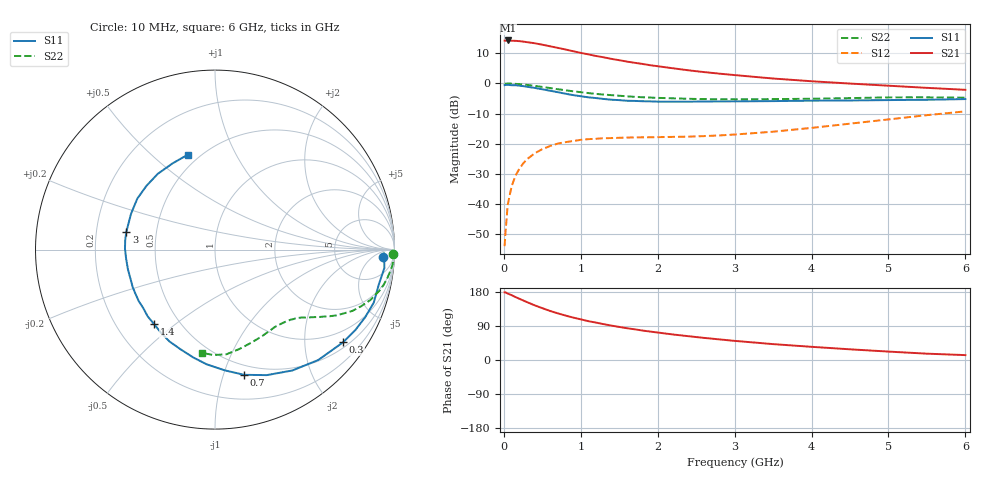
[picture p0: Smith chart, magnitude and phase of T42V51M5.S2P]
! Infineon Technologies  Discrete & RF Semiconductors
! BFR182T
! Si NPN RF Bipolar Junction Transistor in SC75
! VCE = 2.5 V  IC = 1.5 mA
! Common Emitter S-Parameters:  October  1999
# GHz  S  MA  R  50
!  f  S11  S21  S12  S22
! GHz  MAG  ANG  MAG  ANG  MAG  ANG  MAG  ANG
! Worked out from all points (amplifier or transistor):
!   36 points, 10 MHz to 6 GHz, reference 50 ohm
!   highest |S21| = 14.2 dB at 50 MHz (marker M1)
!   |S21| within 3 dB of that: start of sweep to 803.2 MHz
!   unconditionally stable (mu >= 1): 2.156 GHz to 4.436 GHz
!   at 250 MHz: K = 0.11, MSG = 20.2 dB, |S12| = -26.6 dB
!   at 1.4 GHz: K = 0.69, MSG = 13.1 dB, |S12| = -18.1 dB
!   at 6 GHz: K = 0.83, MSG = 3.6 dB, |S12| = -9.3 dB
!   S11 on the Smith chart (normalised r, x): 10 MHz: 22, -14; 300 MHz: 0.64, -2.97; 700 MHz: 0.41, -1.17; 1.4 GHz: 0.36, -0.42; 3 GHz: 0.33, +0.09; 6 GHz: 0.43, +0.66
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0.01  0.9367 -2.4  5.123 178.5  0.002 83.9  0.9908 -1.3
0.02  0.9423 -1.2  5.101 178.6  0.0032 102.5  0.9895 -1.0
0.05  0.9493 -6.2  5.156 175.4  0.0096 88.6  0.9949 -2.5
0.1  0.9333 -11.9  5.102 171.2  0.0195 84.7  0.9927 -4.9
0.15  0.9325 -18.5  5.082 166.3  0.0292 79.6  0.9826 -7.3
0.2  0.9177 -24.2  5.024 161.7  0.0381 78.0  0.9723 -9.6
0.3  0.8814 -35.8  4.835 152.9  0.0552 70.2  0.9453 -13.9
0.4  0.8423 -46.9  4.638 144.3  0.0691 63.9  0.9111 -17.9
0.5  0.7995 -57.4  4.383 136.8  0.0813 59.1  0.8743 -21.1
0.6  0.7564 -67.6  4.131 129.5  0.0916 54.4  0.8387 -24.0
0.7  0.7163 -76.9  3.888 123.2  0.1003 50.7  0.8018 -26.3
0.9  0.6406 -94.2  3.419 112.0  0.1108 44.6  0.7401 -30.1
1.1  0.5873 -109.2  3.031 102.4  0.119 40.6  0.6912 -32.9
1.4  0.5363 -129.2  2.548 90.7  0.124 36.7  0.6384 -36.4
1.8  0.5065 -151.5  2.106 77.8  0.1277 36.0  0.5896 -40.6
2.2  0.4975 -167.4  1.781 67.3  0.1298 37.9  0.5653 -44.8
2.6  0.5016 179.5  1.542 58.4  0.1337 41.6  0.5492 -49.9
3  0.5039 168.7  1.374 50.5  0.142 46.0  0.5451 -54.6
3.5  0.5087 156.8  1.206 41.9  0.1582 51.8  0.5492 -61.7
4.5  0.5216 137.1  0.994 28.2  0.2151 58.4  0.5705 -76.3
5.5  0.5354 116.2  0.844 16.7  0.2976 57.7  0.5876 -90.7
6  0.5498 106.1  0.783 12.9  0.3441 54.9  0.5801 -97.3
